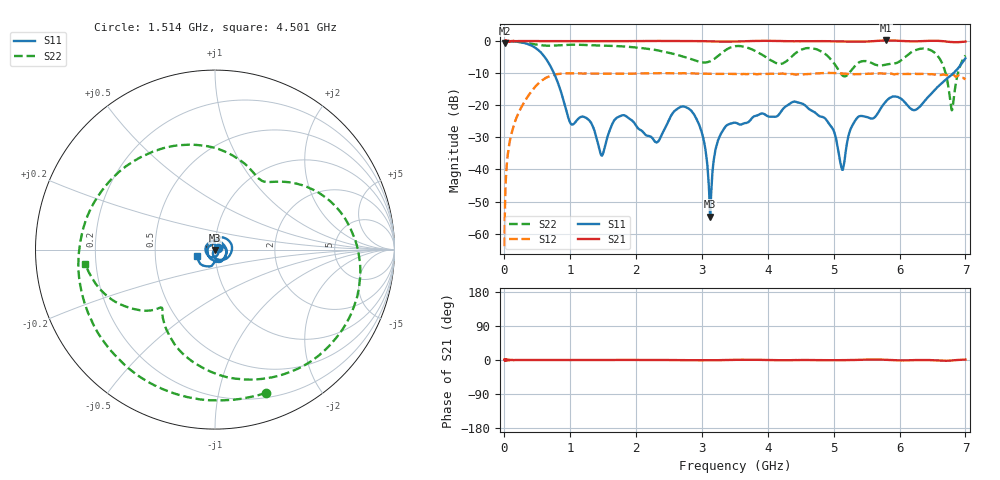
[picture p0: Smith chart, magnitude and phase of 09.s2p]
!Keysight Technologies,N5232A,MY52221221,A.10.65.11
!Date: Wednesday, October 16, 2024 11:56:36
!Correction: S11(Full 2 Port(1,4))
!S41(Full 2 Port(1,4))
!S14(Full 2 Port(1,4))
!S44(Full 2 Port(1,4))
!S2P File: Measurements: S11, S41, S14, S44:
# Hz S  RI  R 50
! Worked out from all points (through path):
!   4000 points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, 2.05 MHz to 7 GHz, reference 50 ohm
!   highest |S21| = 0.19 dB at 5.8 GHz (marker M1); lowest = -0.6 dB at 2.05 MHz (marker M2)
!   lowest |S11| = -54.7 dB at 3.122 GHz (marker M3), VSWR 1.00, Z = 50 - j0.184 ohm
!   |S11| at or under -10 dB: 750.7 MHz to 6.819 GHz (6.068 GHz wide, 160 % of centre)
!   |S22| runs from -21.6 to 0.0 dB; largest |S21 - S12| = 1.3
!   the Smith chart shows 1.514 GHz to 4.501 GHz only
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2049925  -0.9689 0.1508  0.9355 0.0232  0.000131 0.000624  -0.977 0.098
5.979745e7  -0.872 0.4813  1.006 -0.00417  0.00819 0.0185  -0.9761 0.1948
1.805423e8  -0.0365 0.9769  0.9981 -0.000241  0.0601 0.0197  -0.8147 0.5433
3.415354e8  0.8924 0.1671  1 0.00125  0.0874 -0.0979  -0.4299 0.8292
4.867792e8  0.2803 -0.7083  1.001 -0.000889  -0.0806 -0.1879  -0.0499 0.8793
6.320229e8  -0.4585 -0.2585  0.9983 -0.000796  -0.2683 0.0102  0.27 0.8049
1.16925e9  0.0311 0.0586  0.9986 -0.000124  0.1626 -0.2664  0.8454 -0.22
1.477237e9  0.0164 0.00141  0.9971 -0.00025  -0.3113 0.00883  0.3642 -0.7676
1.688978e9  0.0617 -0.00192  0.9965 0.00165  -0.0285 0.3093  -0.1278 -0.8269
2.3347e9  0.00084 0.0272  1.004 0.00106  -0.2873 -0.1297  -0.64 0.3147
2.831679e9  0.069 -0.0464  1.003 -0.01  0.3074 0.0619  0.1196 0.5115
3.122166e9  6.55e-05 -0.00184  0.9896 -0.0129  -0.0556 -0.304  0.303 0.3768
3.5019e9  -0.0525 0.0106  0.9833 0.00841  -0.1238 0.2812  0.7968 -0.2386
3.797637e9  0.0646 -0.0196  1.004 0.0112  0.3072 0.00275  0.0633 -0.71
4.261367e9  -0.0216 -0.0919  0.998 -0.0109  -0.3072 -0.0103  -0.3308 -0.3328
4.66735e9  -0.0805 0.0179  0.9992 -0.00246  0.2723 0.1424  -0.6239 0.4557
5.13108e9  0.00843 -0.00522  0.9863 -0.00689  -0.2823 -0.1358  0.1427 0.2555
5.799551e9  -0.0857 0.0791  1.022 0.00652  0.1827 -0.2519  0.416 -0.1123
5.83455e9  -0.0825 0.0957  1.022 0.00209  0.1182 -0.285  0.414 -0.1483
6.501271e9  0.013 0.1583  1.012 -0.00938  0.2735 0.1331  -0.6353 -0.2835
6.795259e9  0.2879 -0.0846  0.9646 -0.0209  -0.0327 -0.2955  -0.0833 -0.00505
7e9  -0.4444 -0.3045  0.9812 0.0181  -0.2469 0.0488  -0.5943 -0.0492
